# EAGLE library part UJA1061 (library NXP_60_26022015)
Fault-tolerant CAN/LIN fail-safe system basis chip The UJA1061 fail-safe System Basis Chip (SBC) replaces basic discrete components that are common in every Electronic Control Unit (ECU) with a Controller Area Network (CAN) and a Local Interconnect Network (LIN) interface. The fail-safe SBC supports all networking applications that control various power and sensor peripherals by using fault-tolerant CAN as the main network interface and LIN as a local sub-bus. The fail-safe SBC contains the following integrated devices: ISO11898-3 compliant fault-tolerant CAN transceiver, interoperable with TJA1054, TJA1054A and TJA1055 LIN transceiver compliant with LIN 2.0 and SAE J2602, and compatible with LIN 1.3 Advanced independent watchdog Dedicated voltage regulators for microcontroller and CAN transceiver Serial peripheral interface (full duplex) Local wake-up input port Inhibit/limp-home output port In addition to the advantages of integrating these common ECU functions in a single package, the fail-safe SBC offers an intelligent combination of system-specific functions such as: Advanced low-power concept Safe and controlled system start-up behavior Advanced fail-safe system behavior that prevents any conceivable deadlock Detailed status reporting on system and subsystem levels The UJA1061 is designed to be used in combination with a microcontroller that incorporates a CAN controller. The fail-safe SBC ensures that the microcontroller is always started up in a defined manner. In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
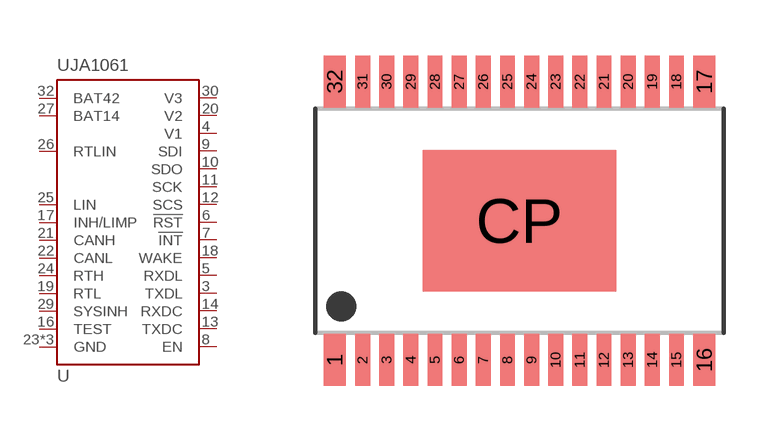
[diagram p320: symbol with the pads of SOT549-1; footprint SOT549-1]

Designator prefix U

## UJA1061TW  [SOT549-1]
3  TXDL  in
4  V1  pwr
5  RXDL  out
6  !RST
7  !INT  out
8  EN  in
9  SDI
10  SDO
11  SCK
12  SCS
13  TXDC  in
14  RXDC  out
16  TEST  in
17  INH/LIMP  out
18  WAKE  in
19  RTL  pas
20  V2  pwr
21  CANH  in
22  CANL  in
23  GND  pwr
24  RTH  pas
25  LIN  in
26  RTLIN  pas
27  BAT14  pwr
29  SYSINH  out
30  V3  pwr
31  GND  pwr
32  BAT42  pwr
CP  GND  pwr

## Footprint SOT549-1 (pad centres in mm)
SOT549-1 HTSSOP32: plastic thermal enhanced thin shrink small outline package; 32 leads;body width 6.1 mm; lead pitch 0.65 mm; exposed die pad JEDEC: MO-153 IEC: -- JEITA: --
smd 0.6 x 1.4: 1 -4.975,-3.75; 16 4.975,-3.75; 17 4.975,3.75; 32 -4.975,3.75
smd 0.4 x 1.4: 2 -4.225,-3.75; 3 -3.575,-3.75; 4 -2.925,-3.75; 5 -2.275,-3.75; 6 -1.625,-3.75; 7 -0.975,-3.75; 8 -0.325,-3.75; 9 0.325,-3.75; 10 0.975,-3.75; 11 1.625,-3.75; 12 2.275,-3.75; 13 2.925,-3.75; 14 3.575,-3.75; 15 4.225,-3.75; 18 4.225,3.75; 19 3.575,3.75; 20 2.925,3.75; 21 2.275,3.75; 22 1.625,3.75; 23 0.975,3.75; 24 0.325,3.75; 25 -0.325,3.75; 26 -0.975,3.75; 27 -1.625,3.75; 28 -2.275,3.75; 29 -2.925,3.75; 30 -3.575,3.75; 31 -4.225,3.75
smd 5.2 x 3.8: CP 0,0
